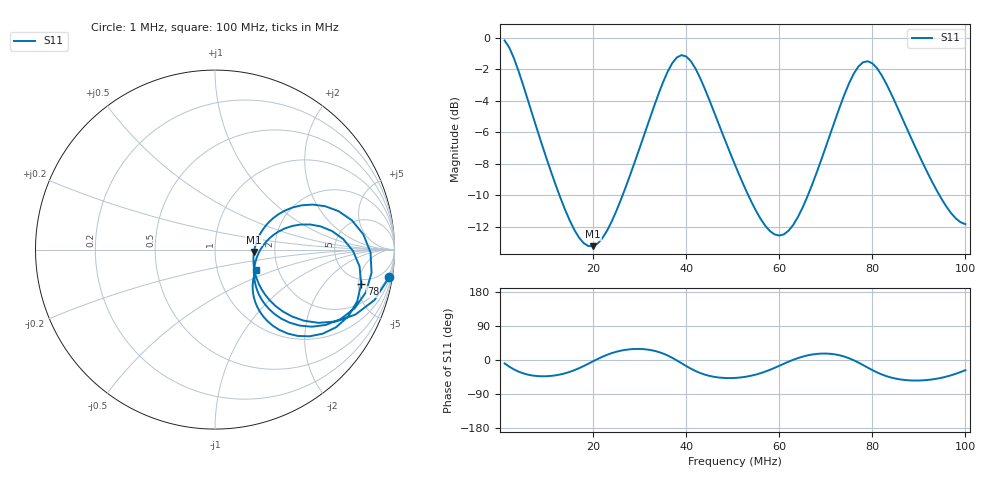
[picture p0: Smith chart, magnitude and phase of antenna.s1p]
# MHz S RI R 50.0
! SimSmith 18.4f
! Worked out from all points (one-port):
!   100 points, 1 MHz to 100 MHz, reference 50 ohm
!   lowest |S11| = -13.2 dB at 20 MHz (marker M1), VSWR 1.56, Z = 77.7 - j2.13 ohm
!   |S11| at or under -10 dB: 12.79 MHz to 26.36 MHz (13.57 MHz wide, 69.3 % of centre); 53.35 MHz to 66.17 MHz (12.82 MHz wide, 21.4 % of centre); 94.42 MHz to end of sweep
!   S11 on the Smith chart (normalised r, x): 1 MHz: 1, -12; 78 MHz: 4.22, -5.39; 100 MHz: 1.53, -0.38
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1  0.9695 -0.1554
3  0.7828 -0.3615
5  0.577 -0.4081
9  0.336 -0.313
14  0.2327 -0.1633
20  0.2173 -0.0131
26  0.2784 0.1279
30  0.3896 0.2174
34  0.6136 0.2416
36  0.7625 0.1631
39  0.8723 -0.1294
41  0.7785 -0.3268
43  0.6171 -0.4197
47  0.3688 -0.3844
51  0.2591 -0.2769
58  0.2189 -0.1061
63  0.2543 0.00209
68  0.3573 0.1023
72  0.5296 0.1399
74  0.6521 0.1034
76  0.7691 -0.0079
78  0.8145 -0.1915
80  0.7427 -0.3717
82  0.6003 -0.4685
85  0.4061 -0.468
88  0.2917 -0.3978
93  0.2172 -0.2687
100  0.228 -0.1159
